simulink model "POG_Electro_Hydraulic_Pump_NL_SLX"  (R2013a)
settings: Solver=ode45  StartTime=0.0  StopTime=10  MaxStep=0.001  RelTol=1e-3
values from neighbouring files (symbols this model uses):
  b_m = 0.02*Nm/(100*rpm)    [POG_Electro_Hydraulic_Pump_NL_SLX_m.m]    (also in POG_Electro_Hydraulic_Pump_Rele_SLX_m.m; POG_Electro_Hydraulic_Pump_SLX_m.m = 1)
  d_0 = (4*mm)^3/sec/(10*atm)    [POG_Electro_Hydraulic_Pump_NL_SLX_m.m]    (also in POG_Electro_Hydraulic_Pump_Rele_SLX_m.m; POG_Electro_Hydraulic_Pump_SLX_m.m = 1)
  F_2_0 = 0    [POG_Electro_Hydraulic_Pump_NL_SLX_m.m]    (also in POG_Electro_Hydraulic_Pump_Rele_SLX_m.m; POG_Electro_Hydraulic_Pump_SLX_m.m)
  J_m = 1*cm^2*1*kg    [POG_Electro_Hydraulic_Pump_NL_SLX_m.m]    (also in POG_Electro_Hydraulic_Pump_Rele_SLX_m.m; POG_Electro_Hydraulic_Pump_SLX_m.m = 1)
  K_m = 0.5    [POG_Electro_Hydraulic_Pump_NL_SLX_m.m]    (also in POG_Electro_Hydraulic_Pump_Rele_SLX_m.m; POG_Electro_Hydraulic_Pump_SLX_m.m = 1; POG_Hydraulic_Clutch_NL_2_SLX_m.m = 16887.5; POG_Hydraulic_Clutch_SS_NL_SLX_m.m = P_a_0*A/(3*cm))
  K_p = 5e-06    [POG_Electro_Hydraulic_Pump_NL_SLX_m.m]    (also in POG_Electro_Hydraulic_Pump_Rele_SLX_m.m; POG_Electro_Hydraulic_Pump_SLX_m.m = 1)
  L_a = 0.3*mHenry    [POG_Electro_Hydraulic_Pump_NL_SLX_m.m]    (also in POG_Electro_Hydraulic_Pump_Rele_SLX_m.m; POG_Electro_Hydraulic_Pump_SLX_m.m = 1)
  P_0 = 5*atm    [POG_Electro_Hydraulic_Pump_NL_SLX_m.m]    (also in POG_Electro_Hydraulic_Pump_Rele_SLX_m.m)
  P_6_0 = 0    [POG_Electro_Hydraulic_Pump_NL_SLX_m.m]    (also in POG_Electro_Hydraulic_Pump_Rele_SLX_m.m; POG_Electro_Hydraulic_Pump_SLX_m.m; POG_Hydraulic_Clutch_SS_NL_SLX_m.m; POG_Hydraulic_Clutch_SS_SLX_m.m)
  Q_0 = (4*cm)^3/sec    [POG_Electro_Hydraulic_Pump_NL_SLX_m.m]    (also in POG_Electro_Hydraulic_Pump_Rele_SLX_m.m)
  R_a = 1*Ohm    [POG_Electro_Hydraulic_Pump_NL_SLX_m.m]    (also in POG_Electro_Hydraulic_Pump_Rele_SLX_m.m; POG_Electro_Hydraulic_Pump_SLX_m.m = 1)
  t_0 = 30*sec    [POG_Electro_Hydraulic_Pump_NL_SLX_m.m]
  Ts = Tfin/Nr_Ts_Points    (= 0.03)    [POG_Electro_Hydraulic_Pump_NL_SLX_m.m]    (also in POG_Electro_Hydraulic_Pump_Rele_SLX_m.m = 0.035; POG_Electro_Hydraulic_Pump_SLX_m.m = 0.005; POG_Hydraulic_Clutch_NL_2_SLX_m.m = 0.0002; POG_Hydraulic_Clutch_SS_NL_SLX_m.m = 0.0002)
  V_0 = (15*cm)^3    [POG_Electro_Hydraulic_Pump_NL_SLX_m.m]    (also in POG_Electro_Hydraulic_Pump_Rele_SLX_m.m)
  V_1_0_0 = 0    [POG_Electro_Hydraulic_Pump_NL_SLX_m.m]    (also in POG_Electro_Hydraulic_Pump_Rele_SLX_m.m; POG_Electro_Hydraulic_Pump_SLX_m.m)
  V_a = 24*Volt    [POG_Electro_Hydraulic_Pump_NL_SLX_m.m]    (also in POG_Electro_Hydraulic_Pump_Rele_SLX_m.m)

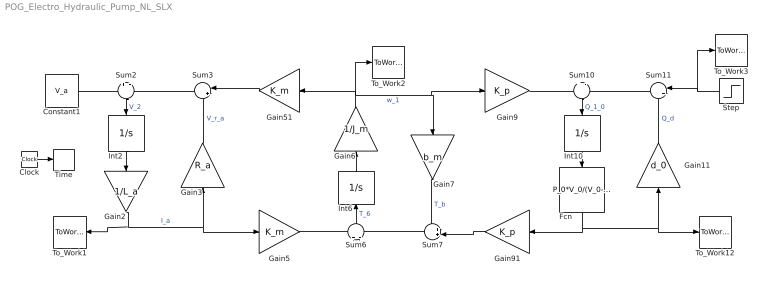
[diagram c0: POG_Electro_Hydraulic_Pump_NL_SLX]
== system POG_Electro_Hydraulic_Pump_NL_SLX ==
  Clock : Clock
  Constant1 : Constant  Value=V_a
  Fcn : Fcn  Expr=P_0*V_0/(V_0-u)
  Gain11 : Gain  Gain=d_0
  Gain2 : Gain  Gain=1/L_a
  Gain3 : Gain  Gain=R_a
  Gain5 : Gain  Gain=K_m
  Gain51 : Gain  Gain=K_m
  Gain6 : Gain  Gain=1/J_m
  Gain7 : Gain  Gain=b_m
  Gain9 : Gain  Gain=K_p
  Gain91 : Gain  Gain=K_p
  Int10 : Integrator  InitialCondition=V_1_0_0  LimitOutput=on  LowerSaturationLimit=0
  Int2 : Integrator  InitialCondition=F_2_0
  Int6 : Integrator  InitialCondition=P_6_0  LimitOutput=on  LowerSaturationLimit=0
  Step : Step  Time=t_0  After=Q_0  SampleTime=0
  Sum10 : Sum  Inputs=+|-
  Sum11 : Sum  Inputs=|++
  Sum2 : Sum  Inputs=+|-
  Sum3 : Sum  Inputs=|++
  Sum6 : Sum  Inputs=+|-
  Sum7 : Sum  Inputs=++|
  Time : ToWorkspace  VariableName=t  SampleTime=Ts
  To_Work1 : ToWorkspace  VariableName=I_a  SampleTime=Ts
  To_Work12 : ToWorkspace  VariableName=P_0  SampleTime=Ts
  To_Work2 : ToWorkspace  VariableName=w_1  SampleTime=Ts
  To_Work3 : ToWorkspace  VariableName=Q_0  SampleTime=Ts
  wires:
  Sum3/1 -> Sum2/2
  Gain2/1 -> To_Work1/1, Gain3/1, Gain5/1  "I_a"
  Sum2/1 -> Int2/1  "V_2"
  Int2/1 -> Gain2/1
  Gain51/1 -> Sum3/1
  Gain3/1 -> Sum3/2  "V_r_a"
  Gain5/1 -> Sum6/1
  Gain6/1 -> To_Work2/1, Gain51/1, Gain7/1, Gain9/1  "w_1"
  Sum7/1 -> Sum6/2
  Sum6/1 -> Int6/1  "T_6"
  Int6/1 -> Gain6/1
  Gain91/1 -> Sum7/2
  Gain7/1 -> Sum7/1  "T_b"
  Gain9/1 -> Sum10/1
  Sum11/1 -> Sum10/2
  Sum10/1 -> Int10/1  "Q_1_0"
  Gain11/1 -> Sum11/2  "Q_d"
  Clock/1 -> Time/1
  Int10/1 -> Fcn/1
  Fcn/1 -> To_Work12/1, Gain11/1, Gain91/1
  Constant1/1 -> Sum2/1
  Step/1 -> To_Work3/1, Sum11/1
